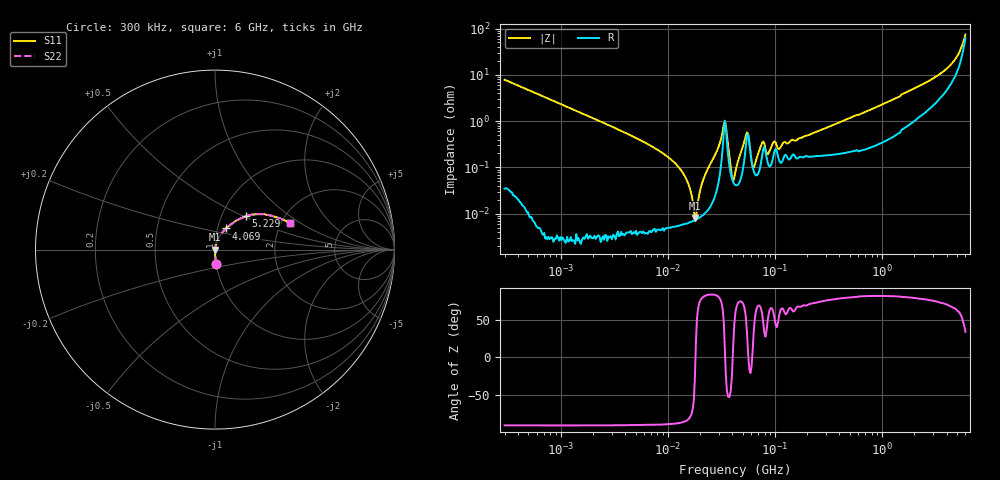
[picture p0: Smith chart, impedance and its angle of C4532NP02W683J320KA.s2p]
! S-Parameter Data Generated by TDK Corporation
! Copyright(C) 2024 TDK Corporation.
! All Rights Reserved.
! TDK P/N: C4532NP02W683J320KA (Multilayer Ceramic Chip Capacitor)
! Property: C=68nF
! Size(LxWxT): 4.5x3.2x3.2mm
! Model Type: s2p (Touchstone File Format Version 1.0)
! Frequency: DC=Yes Start=0.3MHz Stop=6000MHz 402points Log-sweep
! Model Generated on May 28, 2024
! Terms and conditions regarding TDK Simulation Models:
! 1)This simulation model is being provided solely for informational
!  purposes. Please refer to the specifications of the products in
!  terms of detailed characteristics of such products.
! 2)In no event shall TDK Corporation of any of its subsidiaries be
!  liable for any loss or damage arising, directly or indirectly,
!  from any information contained in this simulation model, including,
!  but not limited to loss or damages arising from any inaccuracies,
!  omissions or errors in connection with such information.
! 3)Any and all copyrights on this simulation model are owned by
!  TDK Corporation.  Duplication or redistribution of this simulation
!  model without prior written permission from TDK Corporation
!  is prohibited.
! 4)This simulation model is subject to any modification or change
!  without any prior notice.
! 5)Neither TDK Corporation nor any of its subsidiaries shall make any
!  warranty, express or implied, including but not limited to the
!  correctness, implied warranties of merchantability and fitness for
!  a particular purpose with respect to this simulation models.
! 6)The use of this simulation model shall be deemed to have consented
!  to the terms and conditions hereof.
! Port Assignments:
!  1 ---| |--- 2
! Applicable Conditions:
!  Temperature = 25 degC
!  DC Bias Voltage = 0 V
!  Small Signal Operation
# Hz S MA R 50
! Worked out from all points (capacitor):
!   401 points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, 300 kHz to 6 GHz, reference 50 ohm
!   read as one part in series: C = 67.6 nF near 317.3 kHz
!   lowest |Z| = 8.05 mohm at 17.94 MHz (marker M1)
!   series resonance near 18.15 MHz, so ESL is about 1.1 nH
!   S11 on the Smith chart (normalised r, x): 300 kHz: 1.00, -0.16; 4.069 GHz: 1.10, +0.26; 5.229 GHz: 1.30, +0.52; 6 GHz: 2.24, +0.83
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300000  0.07817 -85.3  0.9966 4.5  0.9966 4.5  0.07817 -85.3
1586297  0.01473 -89.0  0.9999 0.8  0.9999 0.8  0.01473 -89.0
8158352  0.002349 -88.8  1 0.1  1 0.1  0.002349 -88.8
1.432563e7  0.0006689 -84.8  0.9999 0.0  0.9999 0.0  0.0006689 -84.8
1.793851e7  8.051e-05 -25.2  0.9999 0.0  0.9999 0.0  8.051e-05 -25.2
2.142658e7  0.0005424 80.1  0.9999 -0.0  0.9999 -0.0  0.0005424 80.1
2.956217e7  0.002655 80.3  0.9996 -0.2  0.9996 -0.2  0.002655 80.3
3.338291e7  0.008466 44.9  0.994 -0.3  0.994 -0.3  0.008466 44.9
3.49112e7  0.007625 -26.2  0.9932 0.2  0.9932 0.2  0.007625 -26.2
3.973252e7  0.0006285 -23.9  0.9994 0.0  0.9994 0.0  0.0006285 -23.9
4.28954e7  0.0008301 60.2  0.9996 -0.0  0.9996 -0.0  0.0008301 60.2
5.481881e7  0.005688 34.3  0.9953 -0.2  0.9953 -0.2  0.005688 34.3
6.354642e7  0.000995 35.0  0.9992 -0.0  0.9992 -0.0  0.000995 35.0
7.563331e7  0.003293 59.5  0.9983 -0.2  0.9983 -0.2  0.003293 59.5
8.767476e7  0.002085 58.2  0.9989 -0.1  0.9989 -0.1  0.002085 58.2
9.604422e7  0.003361 61.4  0.9984 -0.2  0.9984 -0.2  0.003361 61.4
1.098888e8  0.002499 56.1  0.9986 -0.1  0.9986 -0.1  0.002499 56.1
2.249926e8  0.005438 71.3  0.9983 -0.3  0.9983 -0.3  0.005438 71.3
1.174439e9  0.02685 79.7  0.9955 -1.5  0.9955 -1.5  0.02685 79.7
4.069337e9  0.1325 62.6  0.9464 -7.1  0.9464 -7.1  0.1325 62.6
5.228899e9  0.2527 47.3  0.8492 -12.6  0.8492 -12.6  0.2527 47.3
6e9  0.4458 19.5  0.5985 -14.4  0.5985 -14.4  0.4458 19.5
